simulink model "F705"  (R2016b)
settings: Solver=VariableStepAuto  StartTime=0.0  StopTime=10000  RelTol=1e-3
libraries: simulink x12, sldrtlib x1

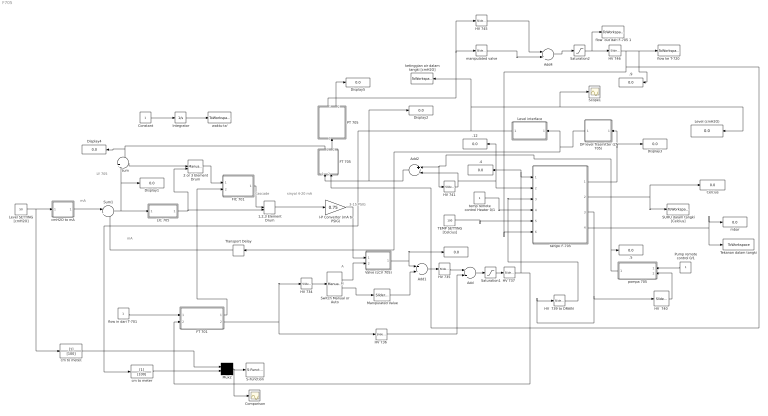
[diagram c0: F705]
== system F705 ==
  note: Cascade
  note: 3-15 PSIG
  note: sinyal 4-20 mA
  note: mA
  note: mA
  note: A
  note: M
  note: LY 705
  .{,4..5,9,12} (5 alike) : Display
  1,2,3 Element Drum : ManualSwitch  RequirementInfo={} %GIDa_980f542c_e3c5_4da0_971b_5ac859e8b983  CurrentSetting=0
  2 or 3 Element Drum : ManualSwitch  RequirementInfo={} %GIDa_bdafc2cf_52f6_4717_81bf_00d028b4eb8e  CurrentSetting=0
  Add : Sum  RequirementInfo={} %GIDa_c7fd6fa8_6156_4bbe_82e1_500e029fe60f
  Add1 : Sum  RequirementInfo={} %GIDa_430d652a_2e23_49c5_a6ef_8d01bf9a6a07
  Add2 : Sum  RequirementInfo={} %GIDa_7aeaae51_2dc6_4cd9_8143_a401e93080b5  Inputs=+-
  Add4 : Sum  RequirementInfo={} %GIDa_5af8e0dc_d8a9_4e06_8e9d_d47c65f90727
  Celcius : Display
  Comparison : Scope
  Constant : Constant  RequirementInfo={} %GIDa_924fa160_b2a7_4ae1_abac_277bfdce7017
  DP level Trasmitter (LT 705) : Subsystem  RequirementInfo={} %GIDa_a84a8026_46b0_43a7_b974_5d67b7de851f
  Display{1..5} (5 alike) : Display
  FIC 701 : Subsystem  RequirementInfo={} %GIDa_47dc6b18_ae06_46a7_bf17_aef032af5448
  FT 701 : Subsystem  RequirementInfo={} %GIDa_e77947e9_91c3_480b_a39f_aac8686264b8
  FT 705 : Subsystem  RequirementInfo={} %GIDa_62322fa3_0e59_4572_9fcf_81ae11d97ec0
  "HV  739 to DRAIN " : simulink/Math Operations/Slider Gain  low=0  gain=0  high=1
  "HV  740 " : simulink/Math Operations/Slider Gain  low=0  gain=1  high=1
  "HV 734 " : simulink/Math Operations/Slider Gain  low=0  gain=1  high=1
  HV 735 : simulink/Math Operations/Slider Gain  low=0  gain=1  high=1
  "HV 736 " : simulink/Math Operations/Slider Gain  low=0  gain=0  high=1
  "HV 737 " : simulink/Math Operations/Slider Gain  low=0  gain=1  high=1
  "HV 741 " : simulink/Math Operations/Slider Gain  low=0  gain=0  high=1
  HV 745 : simulink/Math Operations/Slider Gain  low=0  gain=0  high=1
  "HV 746 " : simulink/Math Operations/Slider Gain  low=0  gain=1  high=1
  I-P Converter (mA to PSIG) : Gain  RequirementInfo={} %GIDa_df3d2db0_99eb_47f4_a1c9_eac6365f6c6a  Gain=0.75
  Integrator : Integrator  RequirementInfo={} %GIDa_83a25a45_bb7d_4185_b062_7bad2054c838
  LIC 705 : Subsystem  RequirementInfo={} %GIDa_ecdd21a2_d821_487f_96c5_fb85d8b0d2ae
  Level (cmH2O) : Display
  Level SETTING [cmH2O] : Constant  RequirementInfo={} %GIDa_b0dee6fe_f864_4748_9d01_491bef8a811d  Value=50
  Level interface : Subsystem
  Manipulated Value : simulink/Math Operations/Slider Gain  low=0  gain=0  high=1
  Mux2 : Mux  RequirementInfo={} %GIDa_9b48d84f_2ec9_4048_959c_1ae083eae352  Inputs=2
  PT 705 : Subsystem  RequirementInfo={} %GIDa_df9374b4_1234_4100_b803_bf93491e16b8
  Pump remote control 0/1 : Constant  RequirementInfo={} %GIDa_56b24d11_95df_4d2d_b70c_011cab4448ee
  S-Function : S-Function  RequirementInfo={} %GIDa_d7104b8f_85b2_4aa7_a9da_7df2386a63e0  FunctionName=animtank  Parameters=1  SFunctionDeploymentMode=off  EnableBusSupport=off
  SUHU dalam tangki [Celcius] : ToWorkspace  VariableName=suhuF705  SampleTime=-1
  Saturation1 : Saturate  RequirementInfo={} %GIDa_34976967_ae65_4c5a_9a44_e363fd89d470  UpperLimit=1  LowerLimit=-99999999999999999999  LinearizeAsGain=off  ZeroCross=off
  Saturation2 : Saturate  RequirementInfo={} %GIDa_302e1a41_6e16_423e_845a_f201a03a66de  UpperLimit=1  LowerLimit=-99999999999999999999  LinearizeAsGain=off  ZeroCross=off
  Scope1 : Scope
  Sum : Sum  RequirementInfo={} %GIDa_14b2a416_5f01_49a8_82b3_3b670bc07b94
  Sum1 : Sum  RequirementInfo={} %GIDa_8cf6189f_0bd7_460f_9ec5_b67d0c72a80a  Inputs=|+-
  Switch Manual or Auto : simulink/Signal Routing/Manual Variant Sink  NumChoices=2  OverrideUsingVariant=V_1
  TEMP SETTING [Celcius] : Constant  RequirementInfo={} %GIDa_8fcc70bf_7ce3_41c6_8138_49938e49a0ae  Value=100
  "Tekanan dalam tangki " : ToWorkspace  VariableName=PressureF705  SampleTime=-1
  Transport Delay : TransportDelay
  Valve (LCV 705) : Subsystem  RequirementInfo={} %GIDa_b8c131ce_1215_44b0_962a_b6fabc49465a
  cm to meter : TransferFcn  RequirementInfo={} %GIDa_489d6a04_48c3_46d1_840e_66fa7c03cbc0  Denominator=[100]
  cm to meter. : TransferFcn  RequirementInfo={} %GIDa_022e435b_aff1_43b5_a887_400e950ce70a  Denominator=[100]
  cmH2O to mA : Subsystem  RequirementInfo={} %GIDa_a20a36d2_4c9c_46bb_b05a_6e2d8adb2ef3
  flow  out dari F-705 1 : ToWorkspace  VariableName=flow_out  SampleTime=-1
  "flow in dari T-701 " : Constant  RequirementInfo={} %GIDa_e76b7a4d_0f41_45a7_9bea_bdb97d502d50
  "flow ke T-720 " : ToWorkspace  VariableName=simout  SaveFormat=Timeseries  SampleTime=-1
  ketinggian air dalam tangki [cmH2O] : ToWorkspace  VariableName=levelF705  SampleTime=-1
  manipulated valve : simulink/Math Operations/Slider Gain  low=0  gain=0.4  high=1
  mbar : Display
  pompa 705 : Subsystem  RequirementInfo={} %GIDa_b18fee99_f8f7_44d7_90f9_778dbbbe63fc
  tangki F-705 : Subsystem  RequirementInfo={} %GIDa_ece88fcb_7ee7_4e20_997f_e499627a89e8
  temp remote control Heater 0/1 : Constant  RequirementInfo={} %GIDa_50c69f00_f857_40cd_94e0_b935a0fbae02
  waktu-ta' : ToWorkspace  VariableName=time  SampleTime=-1
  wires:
  Constant/1 -> Integrator/1
  tangki F-705/2(suhu [Celcius]) -> Celcius/1, SUHU dalam tangki [Celcius]/1
  tangki F-705/3(flow out [Liter/sec]) -> "HV  739 to DRAIN "/1, "HV  740 "/1
  "HV  739 to DRAIN "/1 -> tangki F-705/3(In6)
  "HV 736 "/1 -> Add/2
  HV 735/1 -> Add/1
  TEMP SETTING [Celcius]/1 -> tangki F-705/5(setting)
  FT 705/1(Out1) -> Display4/1, Sum/1
  FIC 701/1(Control) -> 1,2,3 Element Drum/1
  Add/1 -> Saturation1/1
  Mux2/1 -> S-Function/1, Comparison/1
  Pump remote control 0/1/1 -> pompa 705/1(saklar remote)
  Integrator/1 -> waktu-ta'/1
  FT 705/2("Out2 ") -> PT 705/1("In ")
  "HV 741 "/1 -> Add2/2, .12/1, tangki F-705/2(In2)
  "HV 734 "/1 -> Switch Manual or Auto/1
  Switch Manual or Auto/2 -> Manipulated Value/1
  Manipulated Value/1 -> Add1/2
  Add1/1 -> HV 735/1
  FT 701/2(Out2) -> "HV 734 "/1, "HV 736 "/1
  pompa 705/1(Out1) -> .5/1, Add2/1, "HV 741 "/1
  tangki F-705/4(Pressure (Pa)) -> mbar/1, "Tekanan dalam tangki "/1
  cm to meter/1 -> Mux2/2
  cm to meter./1 -> Mux2/1
  Level SETTING [cmH2O]/1 -> cm to meter./1, cmH2O to mA/1(In1)
  cmH2O to mA/1(Out1) -> Sum1/1
  Switch Manual or Auto/1 -> Valve (LCV 705)/2(In2)
  I-P Converter (mA to PSIG)/1 -> Valve (LCV 705)/1(In1)
  Valve (LCV 705)/1(Out1) -> ./1, Add1/1
  LIC 705/1(Control) -> 2 or 3 Element Drum/2, 1,2,3 Element Drum/2
  temp remote control Heater 0/1/1 -> tangki F-705/4(remote on/off)
  Level interface/1(Out1) -> ketinggian air dalam tangki [cmH2O]/1, Scope1/1, Level (cmH2O)/1, cm to meter/1
  PT 705/2(Pressure Flow) -> Display5/1
  "HV  740 "/1 -> pompa 705/2(In2)
  PT 705/1(Out1) -> HV 745/1, manipulated valve/1
  "flow in dari T-701 "/1 -> FT 701/1(In)
  Saturation2/1 -> flow  out dari F-705 1/1, "HV 746 "/1
  Add4/1 -> Saturation2/1
  manipulated valve/1 -> Add4/2
  HV 745/1 -> Add4/1
  "HV 746 "/1 -> FT 705/2(Valve), tangki F-705/6(In3), .9/1, "flow ke T-720 "/1
  DP level Trasmitter (LT 705)/1(Out1) -> Transport Delay/1, Level interface/1(In1)
  Add2/1 -> FT 705/1(In), Display2/1
  Transport Delay/1 -> Sum1/2
  tangki F-705/1(level [cm]) -> Display3/1, DP level Trasmitter (LT 705)/1(In1)
  2 or 3 Element Drum/1 -> FIC 701/1(Set Point)
  Saturation1/1 -> "HV 737 "/1
  1,2,3 Element Drum/1 -> I-P Converter (mA to PSIG)/1
  Sum/1 -> 2 or 3 Element Drum/1
  Sum1/1 -> Display1/1, Sum/2, LIC 705/1(error)
  "HV 737 "/1 -> FT 701/2(valve), .4/1, tangki F-705/1(In1)
  FT 701/1(Out1) -> FIC 701/2(flow in)

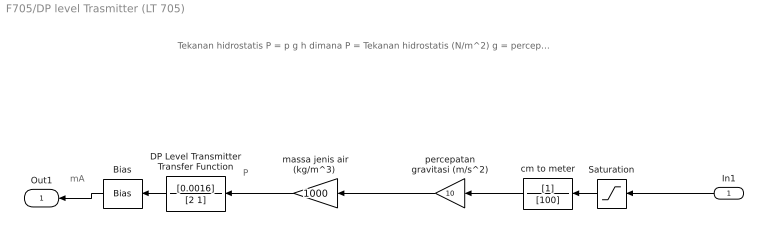
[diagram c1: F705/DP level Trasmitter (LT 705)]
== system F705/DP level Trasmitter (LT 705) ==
  note: P
  note: Tekanan hidrostatis P = p g h dimana P = Tekanan hidrostatis (N/m^2) g = percepatan gravitasi (m/s^2) p = massa jenis air (kg/m^3) h = level fluida
  note: mA
  In1 : Inport  RequirementInfo={} %GIDa_4f80c670_9362_4db7_9b00_538cc1c41416
  Bias : Bias  RequirementInfo={} %GIDa_5fbff64f_7832_4412_9d91_a8b4f3dc1a40  Bias=4
  DP Level Transmitter Transfer Function : TransferFcn  RequirementInfo={} %GIDa_808a6127_73a1_4f3b_8629_1c086189d1f2  Numerator=[0.0016]  Denominator=[2 1]
  Saturation : Saturate  RequirementInfo={} %GIDa_c6edf376_fd32_49be_bfdc_c07c1bae99c1  UpperLimit=100  LowerLimit=0
  cm to meter : TransferFcn  RequirementInfo={} %GIDa_76841945_33ec_46b4_8fbd_d0985e8952ed  Denominator=[100]
  "massa jenis air (kg/m^3) " : Gain  Gain=1000
  percepatan gravitasi (m/s^2) : Gain  Gain=10
  Out1 : Outport  RequirementInfo={} %GIDa_6fa5fe61_9d04_4b16_95a8_0259b73a16a5
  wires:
  Bias/1 -> Out1/1
  DP Level Transmitter Transfer Function/1 -> Bias/1
  Saturation/1 -> cm to meter/1
  cm to meter/1 -> percepatan gravitasi (m/s^2)/1
  percepatan gravitasi (m/s^2)/1 -> "massa jenis air (kg/m^3) "/1
  "massa jenis air (kg/m^3) "/1 -> DP Level Transmitter Transfer Function/1
  In1/1 -> Saturation/1

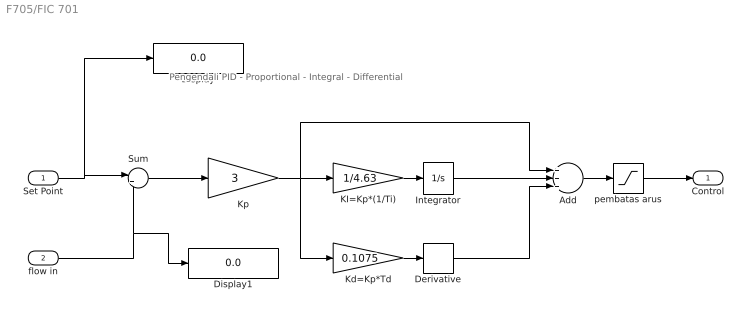
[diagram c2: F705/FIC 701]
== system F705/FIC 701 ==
  note: Pengendali PID - Proportional - Integral - Differential
  Set Point : Inport  RequirementInfo={} %GIDa_b0fab3c2_07d8_47ed_91a1_e495470060ef
  flow in : Inport  RequirementInfo={} %GIDa_4dd8c009_c969_4145_8f79_1f19e3c38768  Port=2
  Add : Sum  RequirementInfo={} %GIDa_1e97b8ae_c40d_4ec3_9219_2518902efba3  Inputs=+++
  Derivative : Derivative  RequirementInfo={} %GIDa_70ab9a75_0a7a_4cf6_8392_a70bb7508225
  Display : Display
  Display1 : Display
  Integrator : Integrator  RequirementInfo={} %GIDa_0c3da3c9_2bb6_4fcc_a20f_4e9bfa180e33  WrappedStateUpperValue=1  WrappedStateLowerValue=0  AbsoluteTolerance=0.000001
  KI=Kp*(1/Ti) : Gain  RequirementInfo={} %GIDa_3a10b322_439d_4a0f_80c4_d72fce9eacda  Gain=1/4.63
  Kd=Kp*Td : Gain  RequirementInfo={} %GIDa_ba25fe83_4212_4623_b273_4efeffd052d5  Gain=0.1075
  Kp : Gain  RequirementInfo={} %GIDa_b942e9b1_6230_457f_b321_ce4571655e46  Gain=3
  Sum : Sum  RequirementInfo={} %GIDa_d1bb208e_1fd0_4e47_aff3_f9c6cfa459ba  Inputs=|+-
  pembatas arus : Saturate  RequirementInfo={} %GIDa_bcf3648f_6a09_4b2c_bc6d_f0f9ab3d20bb  UpperLimit=20  LowerLimit=4  LinearizeAsGain=off  ZeroCross=off
  Control : Outport  RequirementInfo={} %GIDa_efa5d6ef_3b52_4947_a096_e365d12ee2b6
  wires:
  Set Point/1 -> Display/1, Sum/1
  Derivative/1 -> Add/3
  Kd=Kp*Td/1 -> Derivative/1
  KI=Kp*(1/Ti)/1 -> Integrator/1
  Integrator/1 -> Add/2
  Sum/1 -> Kp/1
  Kp/1 -> Add/1, KI=Kp*(1/Ti)/1, Kd=Kp*Td/1
  flow in/1 -> Display1/1, Sum/2
  Add/1 -> pembatas arus/1
  pembatas arus/1 -> Control/1

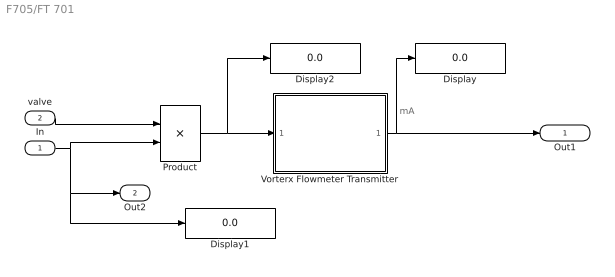
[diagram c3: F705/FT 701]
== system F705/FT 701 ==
  note: mA
  In : Inport  RequirementInfo={} %GIDa_716ed75a_19f1_4e87_8fd9_ecdccbd7f266
  valve : Inport  RequirementInfo={} %GIDa_230247e2_c477_4d24_9ea3_f282d17bc786  Port=2
  Display : Display
  Display1 : Display
  Display2 : Display
  Product : Product  RequirementInfo={} %GIDa_0f950e1b_6a03_46f8_b4f6_1be5aecbfbb5
  Vorterx Flowmeter Transmitter : Subsystem  RequirementInfo={} %GIDa_a876f043_ab4d_4b3a_b757_7d6ece9ec400
  Out1 : Outport  RequirementInfo={} %GIDa_0175ceae_9a6e_4547_90ae_6849443ca355
  Out2 : Outport  RequirementInfo={} %GIDa_d790bc43_a55a_4c07_bff8_18ba5bf84909  Port=2
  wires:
  valve/1 -> Product/1
  In/1 -> Display1/1, Out2/1, Product/2
  Vorterx Flowmeter Transmitter/1(Out1) -> Out1/1, Display/1
  Product/1 -> Display2/1, Vorterx Flowmeter Transmitter/1(In1)

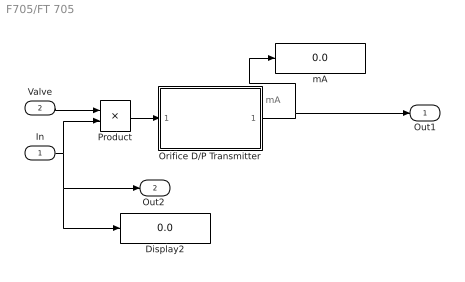
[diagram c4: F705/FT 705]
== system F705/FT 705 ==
  note: mA
  In : Inport  RequirementInfo={} %GIDa_404fc8e2_91c3_4800_bf44_fc00c912c336
  Valve : Inport  RequirementInfo={} %GIDa_95875d8d_45fa_4d2c_8149_751ebdd7b960  Port=2
  Display2 : Display
  Orifice D/P Transmitter : Subsystem  RequirementInfo={} %GIDa_500a6f29_080f_4f6e_a546_92cb3a08a525
  Product : Product
  mA : Display
  Out1 : Outport  RequirementInfo={} %GIDa_4dccba8b_6749_4e81_b118_20321c4423f2
  "Out2 " : Outport  RequirementInfo={} %GIDa_05ed0961_4b54_46e9_8ac6_92b81f5e989c  Port=2
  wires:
  In/1 -> Product/2, Display2/1, "Out2 "/1
  Orifice D/P Transmitter/1(Out1) -> mA/1, Out1/1
  Valve/1 -> Product/1
  Product/1 -> Orifice D/P Transmitter/1(In1)

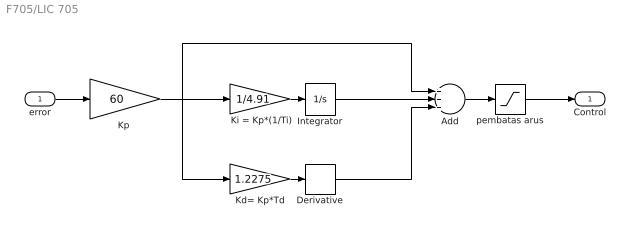
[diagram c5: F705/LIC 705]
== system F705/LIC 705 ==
  error : Inport  RequirementInfo={} %GIDa_6d8e38b2_3745_448e_8017_853de8079433
  " Ki = Kp*(1/Ti)" : Gain  RequirementInfo={} %GIDa_e69da03a_a0da_4704_bb54_0798b217f956  Gain=1/4.91
  Add : Sum  RequirementInfo={} %GIDa_7bfcf71b_5572_4f84_a8c6_bd6bf2c96ae6  Inputs=+++
  Derivative : Derivative  RequirementInfo={} %GIDa_7f956c3f_e6ae_4d53_856a_6020102b4141
  Integrator : Integrator  RequirementInfo={} %GIDa_213e6744_b9fd_4605_bac6_1177a5d9195d  WrappedStateUpperValue=1  WrappedStateLowerValue=0  AbsoluteTolerance=0.000001
  Kd= Kp*Td : Gain  RequirementInfo={} %GIDa_8fb87115_65ca_4557_9584_410990ceb832  Gain=1.2275
  "Kp " : Gain  RequirementInfo={} %GIDa_640f1607_9d17_4811_8483_188dee7691ef  Gain=60
  pembatas arus : Saturate  RequirementInfo={} %GIDa_705c5f2f_4e80_4692_a01a_272046ac20b7  UpperLimit=20  LowerLimit=4  LinearizeAsGain=off  ZeroCross=off
  Control : Outport  RequirementInfo={} %GIDa_8820d1ad_dc0e_4bab_9293_6ed03fa2ccb6
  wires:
  Derivative/1 -> Add/3
  Kd= Kp*Td/1 -> Derivative/1
  " Ki = Kp*(1/Ti)"/1 -> Integrator/1
  Integrator/1 -> Add/2
  error/1 -> "Kp "/1
  "Kp "/1 -> Add/1, " Ki = Kp*(1/Ti)"/1, Kd= Kp*Td/1
  Add/1 -> pembatas arus/1
  pembatas arus/1 -> Control/1

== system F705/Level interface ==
  In1 : Inport
  Bias : Bias  RequirementInfo={} %GIDa_589ebe2f_df52_44e7_866e_ee1e8d6ceade  Bias=-4
  Transfer Fcn : TransferFcn  Denominator=[0.16]
  Out1 : Outport
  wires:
  In1/1 -> Bias/1
  Transfer Fcn/1 -> Out1/1
  Bias/1 -> Transfer Fcn/1

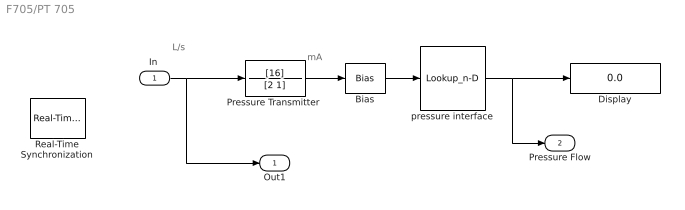
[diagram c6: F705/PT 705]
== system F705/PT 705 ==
  note: L/s
  note: mA
  "In " : Inport  RequirementInfo={} %GIDa_ed38d12a_45c5_4e04_b2ef_af6cf30e9bd9
  Bias : Bias  RequirementInfo={} %GIDa_9fcaf6f5_b79d_4fba_9047_14212e301499  Bias=4
  Display : Display
  "Pressure Transmitter " : TransferFcn  RequirementInfo={} %GIDa_3436b8e0_8631_408d_a4f1_07208803dcc0  Numerator=[16]  Denominator=[2 1]
  Real-Time Synchronization : sldrtlib/Real-Time Synchronization  SampleTime=1  MaxMissedTicks=10  ShowMissedTicks=off  YieldWhenWaiting=off
  pressure interface : Lookup_n-D  NumberOfTableDimensions=1  BreakpointsForDimension1=[4,5,6,7,8,9,10,11,12,13,14,15,16,17,18,19,20]  Table=[0,1.875,3.75,5.625,7.5,9.375,11.25,13.125,15,16.875,18.75,20.625,22.5,24.375,26.25,28.125,30]  InternalRulePriority=Speed  RndMeth=Simplest
  Out1 : Outport  RequirementInfo={} %GIDa_b303f539_540f_44cc_8f69_73332774cf5f
  Pressure Flow : Outport  RequirementInfo={} %GIDa_2528cfde_cd49_4a36_802a_edfb8f764deb  Port=2
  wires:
  "Pressure Transmitter "/1 -> Bias/1
  "In "/1 -> "Pressure Transmitter "/1, Out1/1
  Bias/1 -> pressure interface/1
  pressure interface/1 -> Pressure Flow/1, Display/1

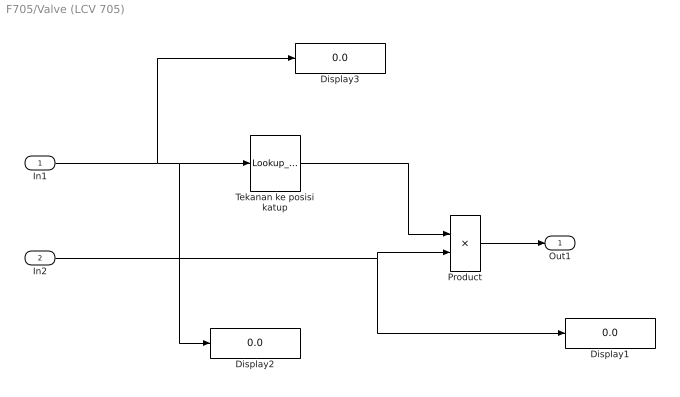
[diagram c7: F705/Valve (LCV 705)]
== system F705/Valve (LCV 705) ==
  In1 : Inport  RequirementInfo={} %GIDa_68acfe16_5018_41ad_bb22_6e90cc35faec
  In2 : Inport  RequirementInfo={} %GIDa_b4cb757c_c2a3_467f_b272_bcde135826d0  Port=2
  Display1 : Display
  Display2 : Display
  Display3 : Display
  Product : Product  RequirementInfo={} %GIDa_90b649b9_9d42_408e_b265_3f135f991b21
  Tekanan ke posisi katup : Lookup_n-D  RequirementInfo={} %GIDa_88c65955_9d2c_460c_8dd3_ab0c9b94b05e  NumberOfTableDimensions=1  BreakpointsForDimension1=single([3,4,5,6,7,8,9,10,11,12,13,14,15]);  Table=single([0,0.08333333,0.16666666,0.25,0.33333333,0.41666666,0.5,0.58333333,0.66666666,0.75,0.83333333,0.91666666,1]);  InternalRulePriority=Speed  RndMeth=Simplest
  Out1 : Outport  RequirementInfo={} %GIDa_a4536907_4416_49c7_810f_faa02db84965
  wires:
  In2/1 -> Display1/1, Product/2
  Product/1 -> Out1/1
  In1/1 -> Display3/1, Display2/1, Tekanan ke posisi katup/1
  Tekanan ke posisi katup/1 -> Product/1

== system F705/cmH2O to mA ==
  note: mA
  In1 : Inport  RequirementInfo={} %GIDa_8254bc63_fd78_496f_9996_28d34f190487
  Bias : Bias  RequirementInfo={} %GIDa_cc70ba2c_b8e2_4bdb_8724_61be6dee9fa1  Bias=4
  Gain : Gain  RequirementInfo={} %GIDa_0834c4c8_c3a3_45bd_aa23_85ff76ed7596  Gain=0.16
  Out1 : Outport  RequirementInfo={} %GIDa_11c030b9_7fb0_44fb_8588_4185fefdfd53
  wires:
  In1/1 -> Gain/1
  Gain/1 -> Bias/1
  Bias/1 -> Out1/1

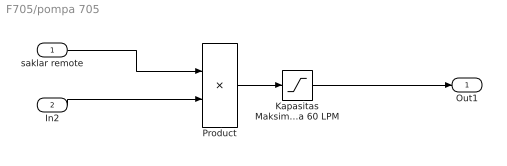
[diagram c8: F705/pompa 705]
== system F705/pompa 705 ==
  saklar remote : Inport  RequirementInfo={} %GIDa_268dfa0e_25db_4a16_8228_501bdf0b6bdc
  In2 : Inport  RequirementInfo={} %GIDa_bbf477b2_b7e9_44bc_8907_a047c8d5c446  Port=2
  Kapasitas Maksimum Pompa 60 LPM : Saturate  RequirementInfo={} %GIDa_a08010ca_8263_42f7_bc9b_4cb1ed9342fe  UpperLimit=1  LowerLimit=-9999999999999999999999999999999999999999  LinearizeAsGain=off  ZeroCross=off
  Product : Product  RequirementInfo={} %GIDa_b00c0488_9eb8_4888_8a8e_d31f7b8799d3
  Out1 : Outport  RequirementInfo={} %GIDa_3e0205ae_ce0b_4b64_acdb_4cd33bd326c7
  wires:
  Product/1 -> Kapasitas Maksimum Pompa 60 LPM/1
  In2/1 -> Product/2
  saklar remote/1 -> Product/1
  Kapasitas Maksimum Pompa 60 LPM/1 -> Out1/1

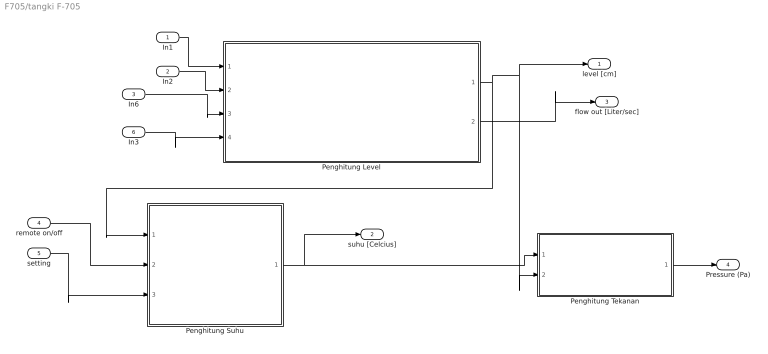
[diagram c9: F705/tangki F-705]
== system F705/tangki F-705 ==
  In1 : Inport  RequirementInfo={} %GIDa_85515634_4662_4253_b92c_74cb03839840
  In2 : Inport  RequirementInfo={} %GIDa_a913a49c_a44d_4a46_8383_7b1a68edbef0  Port=2
  In6 : Inport  RequirementInfo={} %GIDa_2246ca63_b8c4_4b59_9067_2978b757a582  Port=3
  remote on/off : Inport  RequirementInfo={} %GIDa_4bee1f29_9d60_4ad4_b0b4_0c282e461e29  Port=4
  setting : Inport  RequirementInfo={} %GIDa_8b63f729_085c_4801_8cb8_ce72f5b7c9f4  Port=5
  In3 : Inport  RequirementInfo={} %GIDa_d7e9f3ba_24bc_48bd_915b_b241cc8ecfda  Port=6
  Penghitung Level : Subsystem  RequirementInfo={} %GIDa_97f18464_5942_4876_ae07_b78c7015ac08
  Penghitung Suhu : Subsystem  RequirementInfo={} %GIDa_a2eaa51c_c4e3_477b_9a7b_c50059d0c719
  Penghitung Tekanan : Subsystem  RequirementInfo={} %GIDa_bcb36fdf_897b_49c0_a7d4_11c7b023a67c
  level [cm] : Outport  RequirementInfo={} %GIDa_77a68ff4_bf90_44a4_935a_fa74adf82e0c
  suhu [Celcius] : Outport  RequirementInfo={} %GIDa_d3be4350_b1f8_49ea_9576_4617f54eba14  Port=2
  flow out [Liter/sec] : Outport  RequirementInfo={} %GIDa_e3ebabc5_2c2c_41c9_9a68_4d87ed112b13  Port=3
  Pressure (Pa) : Outport  RequirementInfo={} %GIDa_3f4a3c5c_f715_447f_a863_f6abc0ff06f2  Port=4
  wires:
  Penghitung Suhu/1(suhu) -> suhu [Celcius]/1, Penghitung Tekanan/1(Suhu)
  In2/1 -> Penghitung Level/2(Dari Pompa lewat HV-741)
  In6/1 -> Penghitung Level/3(Drain)
  Penghitung Level/1(level [cmH2O]) -> level [cm]/1, Penghitung Tekanan/2(Level), Penghitung Suhu/1(level[cm])
  remote on/off/1 -> Penghitung Suhu/2(Remote Heater)
  In1/1 -> Penghitung Level/1(dari T-701)
  In3/1 -> Penghitung Level/4(Pompa 705)
  Penghitung Level/2(debit out (Liter/sec)) -> flow out [Liter/sec]/1
  setting/1 -> Penghitung Suhu/3(Set Point)
  Penghitung Tekanan/1(Pressure tangki (mbar)) -> Pressure (Pa)/1

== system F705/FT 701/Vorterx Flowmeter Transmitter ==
  note: mA
  In1 : Inport  RequirementInfo={} %GIDa_678609eb_e02c_441a_9dc0_97b0472d8144
  Bias : Bias  RequirementInfo={} %GIDa_703a9e3c_f886_4603_b782_0bf3f8227f68  Bias=4
  Vortex Flowmeter Transmitter Transfer Function : TransferFcn  RequirementInfo={} %GIDa_730bb598_0391_4812_9619_57cea0a7dee6  Numerator=[16]  Denominator=[4 1]
  Out1 : Outport  RequirementInfo={} %GIDa_aaee8f26_3184_423e_a188_077b8c8caf9f
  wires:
  Vortex Flowmeter Transmitter Transfer Function/1 -> Bias/1
  Bias/1 -> Out1/1
  In1/1 -> Vortex Flowmeter Transmitter Transfer Function/1

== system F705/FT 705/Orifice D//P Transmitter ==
  In1 : Inport  RequirementInfo={} %GIDa_c017005f_6fab_4ee6_a132_fd49cbfe2310
  Bias : Bias  RequirementInfo={} %GIDa_e677cbcd_2831_47f9_908a_0e51e9fff569  Bias=4
  Orifice DP Flowmeter Transmitter Transfer Function : TransferFcn  RequirementInfo={} %GIDa_27d93213_c8c3_46ef_a334_83aa21ba1e3d  Numerator=[16]  Denominator=[2 1]
  Out1 : Outport  RequirementInfo={} %GIDa_37e754d4_d1f6_4396_b99c_b299c777b81a
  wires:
  Bias/1 -> Out1/1
  Orifice DP Flowmeter Transmitter Transfer Function/1 -> Bias/1
  In1/1 -> Orifice DP Flowmeter Transmitter Transfer Function/1

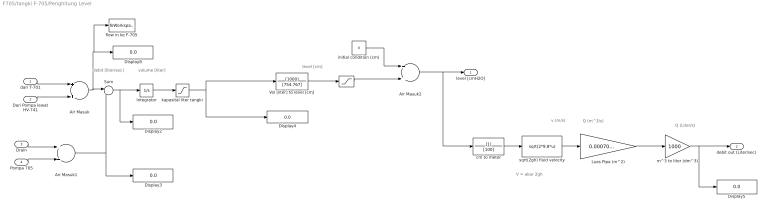
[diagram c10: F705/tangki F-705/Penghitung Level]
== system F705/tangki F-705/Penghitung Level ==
  note: V = akar 2gh
  note: Q (Liter/s)
  note: Q (m^3/s)
  note: v (m/s)
  note: debit [liter/sec]
  note: level [cm]
  note: volume [liter]
  dari T-701 : Inport  RequirementInfo={} %GIDa_c65f6753_e8f0_4630_b1d2_d884af79a199
  Dari Pompa lewat HV-741 : Inport  RequirementInfo={} %GIDa_fc0150cc_5002_4fa2_a6b9_49191c4481e6  Port=2
  Drain : Inport  RequirementInfo={} %GIDa_ae89c716_532d_48be_9893_5c428c75a659  Port=3
  Pompa 705 : Inport  RequirementInfo={} %GIDa_df2140be_7e08_47d9_9c82_f4a59c2ae3f6  Port=4
  . : Saturate  RequirementInfo={} %GIDa_54b3a901_0ab2_4439_abd9_bb0ec5550532  UpperLimit=119.5  LowerLimit=-999999999999999999999999999999999999999999999999999  LinearizeAsGain=off  ZeroCross=off
  Air Masuk : Sum  RequirementInfo={} %GIDa_d4e6bf9b_1e62_4201_b132_a3032806f737
  Air Masuk1 : Sum  RequirementInfo={} %GIDa_cd94d44b_924b_4337_accc_f6d2e33b1381
  Air Masuk2 : Sum  RequirementInfo={} %GIDa_1f4c05a7_ec00_42d0_9add_5e9083b01e47
  Display{2..5,8} (5 alike) : Display
  Integrator : Integrator  RequirementInfo={} %GIDa_87842f1e_d65f_4519_a0dd_042002f68c4d
  Luas Pipa (m^2) : Gain  RequirementInfo={} %GIDa_411c5f22_d837_4ea4_b771_dcc9a33ae0ef  Gain=0.000706858347
  Sum : Sum  RequirementInfo={} %GIDa_5d77d671_2315_480b_b505_b388c8dadcfb  Inputs=|+-
  Vol [liter] to level [cm] : TransferFcn  RequirementInfo={} %GIDa_77694d0d_8775_4e37_a832_4f4063e56a58  Numerator=[1000]  Denominator=[754.767]
  cm to meter : TransferFcn  RequirementInfo={} %GIDa_04395537_007e_4c8c_95a3_d78ddf15ff93  Denominator=[100]
  "flow in ke F-705 " : ToWorkspace  VariableName=flow_in  SampleTime=-1
  "initial condition (cm) " : Constant  Value=0
  kapasital liter tangki : Saturate  RequirementInfo={} %GIDa_84c55fd7_ded1_4924_a33b_0ba97317ca9e  UpperLimit=100  LowerLimit=-99999999999999999999999999999999999999999999999999  LinearizeAsGain=off  ZeroCross=off
  m^3 to liter (dm^3) : Gain  RequirementInfo={} %GIDa_7653e8eb_9ac4_4175_af70_28424efe7908  Gain=1000
  sqrt(2gh) fluid velocity : Fcn  RequirementInfo={} %GIDa_e05a83f4_1597_4967_bc69_3ac066331f28  Expr=sqrt(2*9.8*u)
  level [cmH2O] : Outport  RequirementInfo="{'linktype_rmi_simulink' 'D' ':376' 'true' 'D/Lamp  (SubSystem)' '' } %GIDa_5d4fb5c8_aef1_4d30_ac98_30f6286ac0b0"
  debit out (Liter/sec) : Outport  RequirementInfo={} %GIDa_a7e5f6d6_5d50_4d5a_b337_e60b99e73b88  Port=2
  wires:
  Sum/1 -> Display2/1, Integrator/1
  Air Masuk/1 -> Sum/1, "flow in ke F-705 "/1, Display8/1
  Dari Pompa lewat HV-741/1 -> Air Masuk/2
  dari T-701/1 -> Air Masuk/1
  Integrator/1 -> kapasital liter tangki/1
  Drain/1 -> Air Masuk1/1
  Air Masuk1/1 -> Sum/2, Display3/1
  sqrt(2gh) fluid velocity/1 -> Luas Pipa (m^2)/1
  Luas Pipa (m^2)/1 -> m^3 to liter (dm^3)/1
  Pompa 705/1 -> Air Masuk1/2
  cm to meter/1 -> sqrt(2gh) fluid velocity/1
  kapasital liter tangki/1 -> Vol [liter] to level [cm]/1, Display4/1
  Vol [liter] to level [cm]/1 -> ./1
  m^3 to liter (dm^3)/1 -> Display5/1, debit out (Liter/sec)/1
  ./1 -> Air Masuk2/2
  Air Masuk2/1 -> cm to meter/1, level [cmH2O]/1
  "initial condition (cm) "/1 -> Air Masuk2/1

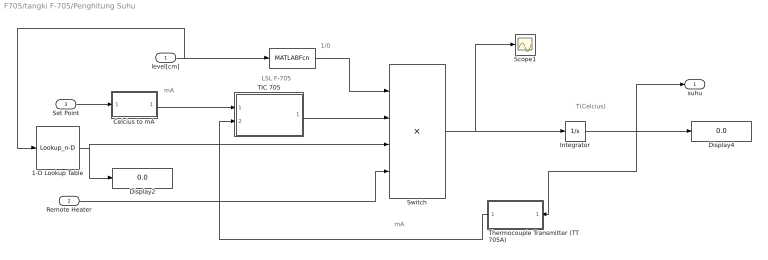
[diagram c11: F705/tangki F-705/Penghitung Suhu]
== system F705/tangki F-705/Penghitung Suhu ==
  note: mA
  note: mA
  note: T(Celcius)
  note: LSL F-705
  note: 1/0
  level[cm] : Inport  RequirementInfo={} %GIDa_b7ffd82a_15ed_4e5e_8a60_4e6a5822e138
  Remote Heater : Inport  RequirementInfo={} %GIDa_d83ed7be_1f0c_4871_9373_09444e220b47  Port=2
  Set Point : Inport  RequirementInfo={} %GIDa_6436afb1_2948_4352_9d49_1c4604274298  Port=3
  " " : MATLABFcn  RequirementInfo="{'linktype_rmi_simulink' 'D' ':376' 'true' 'D/Lamp  (SubSystem)' '' } %GIDa_dd4a015e_e96f_4f79_ad44_2c4b5cf474a1"  MATLABFcn=LSL705
  1-D Lookup Table : Lookup_n-D  NumberOfTableDimensions=1  BreakpointsForDimension1=[20,30,40,50]  Table=[0.1204,0.08678,0.06899,0.05397]  InternalRulePriority=Speed  RndMeth=Simplest
  Celcius to mA : Subsystem  RequirementInfo={} %GIDa_8efdd625_884a_4c63_868a_44d367e44511
  Display2 : Display
  Display4 : Display
  Integrator : Integrator  RequirementInfo={} %GIDa_cd4c95bc_218f_4784_b80d_0dbed389e141  InitialCondition=31.4
  Scope1 : Scope
  Switch : Product  RequirementInfo={} %GIDa_6577b0c3_d5f6_42c4_b5a4_029077d4e36c  Inputs=4
  TIC 705 : Subsystem  RequirementInfo={} %GIDa_a9bf4c55_676b_44a7_b111_bd1e19c22f9f
  Thermocouple Transmitter (TT 705A) : Subsystem  RequirementInfo={} %GIDa_d9cb32aa_fc91_4ffc_a42e_bcffe28f5e31
  suhu : Outport  RequirementInfo={} %GIDa_ea196fef_df6d_47dc_9f73_9dee72b243a7
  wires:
  level[cm]/1 -> 1-D Lookup Table/1, " "/1
  Switch/1 -> Scope1/1, Integrator/1
  Remote Heater/1 -> Switch/4
  TIC 705/1(Out1) -> Switch/2
  " "/1 -> Switch/1
  1-D Lookup Table/1 -> Display2/1, Switch/3
  Thermocouple Transmitter (TT 705A)/1(Out2) -> TIC 705/2(In3)
  Set Point/1 -> Celcius to mA/1(In1)
  Celcius to mA/1(Out1) -> TIC 705/1(In2)
  Integrator/1 -> Thermocouple Transmitter (TT 705A)/1(In2), suhu/1, Display4/1

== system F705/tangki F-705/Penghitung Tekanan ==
  Suhu : Inport  RequirementInfo={} %GIDa_ddf55136_42ce_483a_9da6_6fef0310dbfb
  Level : Inport  RequirementInfo={} %GIDa_56a105ca_a29c_447f_a322_02cee1bfd1b5  Port=2
  Bourdon Tube : Lookup_n-D  RequirementInfo={} %GIDa_ddde6720_9a6b_4ea5_8b4f_7c34fcde0cfa  BreakpointsForDimension1=[28,29,30,31,32,33,34,35,36,37,38,39,40,41,42,43,44,45,46,47,48,49,50,51,52,53,54,55,56,57,58,59,60,61,62,63,64,65,66,67,68,69,70,71,72,73,74,75,76,77,78,79,80,81,82,83,84,85,86,87,88,89,90,91,92,93,94,95,96,97,98,99,100]  BreakpointsForDimension2=[30,40,50]  Table=reshape([0,0,0,0,0,0,0,0,0,0,0,0,0,0,0,0,0,0,0,0,0,0,0,0,0,0,0,0,0,0,0,0,0,0,0,0,0,0,0,0,0,0,0,0,0,0,0,0,1,3,9,10,10,11,12,13,14,14,15,15,16,18,20,20,22,24,25,26,27,28,29,29,30,0,0,0,0,0,0,0,0,0,0,0,0,0,0,0,0,0,0,0,0,0,0,0,0,0,0,0,0,0,0,0,0,0,0,0,0,0,0,0,0,0,0,0,0,0,0,1,5,8,7,10,10,11,12,13,14,14,15,16,17,18,20,21,22,24,25,25,27,29,30,31,31,32,0,0,0,0,0,0,0,0,0,0,0,0,0,0,0,0,0,0,0,0,0,0,0,0,0,0,0,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  InternalRulePriority=Speed  RndMeth=Simplest
  Display1 : Display
  Pressure tangki (mbar) : Outport  RequirementInfo={} %GIDa_976ca7db_6240_4b85_b81c_f417ffed3128
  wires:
  Suhu/1 -> Bourdon Tube/1
  Level/1 -> Bourdon Tube/2
  Bourdon Tube/1 -> Display1/1, Pressure tangki (mbar)/1

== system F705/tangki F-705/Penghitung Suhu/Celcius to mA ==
  In1 : Inport  RequirementInfo={} %GIDa_576f8054_ff83_4d87_b38a_fc9a9f469c13
  Add : Sum  RequirementInfo={} %GIDa_6176f9af_c43b_41ae_8ca0_19c03e431ad4
  initial condition (mA) : Constant  RequirementInfo={} %GIDa_49dc0110_73cc_419e_98b3_921618199f0f  Value=4
  to mA : Gain  RequirementInfo={} %GIDa_50039649_2a02_4dd6_b739_4be1eab27110  Gain=0.16
  Out1 : Outport  RequirementInfo={} %GIDa_4e360bf2_9221_49dd_acb2_7cf980cfed9d
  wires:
  In1/1 -> to mA/1
  to mA/1 -> Add/1
  Add/1 -> Out1/1
  initial condition (mA)/1 -> Add/2

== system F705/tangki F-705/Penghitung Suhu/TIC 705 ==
  note: 1/0
  In2 : Inport  RequirementInfo={} %GIDa_e8a8c583_0914_4ba5_9724_fea1e8bd28d6
  In3 : Inport  RequirementInfo={} %GIDa_2a31af98_8726_4efc_8be3_652eca402edf  Port=2
  ON/OFF Controller : MATLABFcn  RequirementInfo={} %GIDa_c08efdae_68d2_48bc_bdd0_31b09ca989ee  MATLABFcn=TM
  Sum1 : Sum  RequirementInfo={} %GIDa_90c2ddf8_11fc_4eab_afdc_576db9bccae6  Inputs=|+-
  Out1 : Outport  RequirementInfo={} %GIDa_a1ec9056_103c_445a_87c9_7a717e1fa746
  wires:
  In3/1 -> Sum1/2
  Sum1/1 -> ON/OFF Controller/1
  In2/1 -> Sum1/1
  ON/OFF Controller/1 -> Out1/1

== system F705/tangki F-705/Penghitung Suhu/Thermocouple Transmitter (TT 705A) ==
  In2 : Inport  RequirementInfo={} %GIDa_cf1a7155_e8a0_40f3_9dd0_83a6d081848b
  Bias : Bias  RequirementInfo={} %GIDa_6f8b0347_8084_4eb8_9c24_72527ca53dbf  Bias=4
  Thermocouple Sensor : TransferFcn  RequirementInfo={} %GIDa_ed14c7c0_2d55_4630_b48a_d8fa7ef38e21  Numerator=[0.16]  Denominator=[1 1]
  Out2 : Outport  RequirementInfo={} %GIDa_cd9f88dc_fd44_4eb9_9e51_6a261f02c5fc
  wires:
  Bias/1 -> Out2/1
  In2/1 -> Thermocouple Sensor/1
  Thermocouple Sensor/1 -> Bias/1
